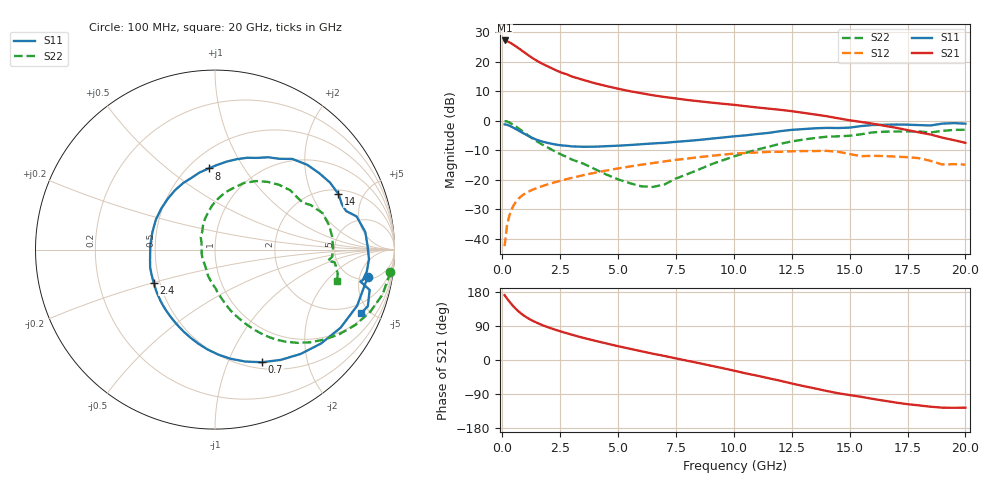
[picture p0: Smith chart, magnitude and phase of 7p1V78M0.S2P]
! Infineon Technologies  Discrete & RF Semiconductors
! bfp620
! VCE =  1.7 V,  IC =  8.0 mA
! Common Emitter S-Parameters:  Sep 2002
# GHz  S  MA  R  50
!  f  S11  S21  S12  S22
! GHz  MAG  ANG  MAG  ANG  MAG  ANG  MAG  ANG
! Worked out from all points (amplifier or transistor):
!   59 points, 100 MHz to 20 GHz, reference 50 ohm
!   highest |S21| = 27.1 dB at 100 MHz (marker M1)
!   |S21| within 3 dB of that: start of sweep to 769.9 MHz
!   unconditionally stable (mu >= 1): 4.315 GHz to 10.93 GHz; 17.11 GHz to end of sweep
!   at 1 GHz: K = 0.43, MSG = 23.7 dB, |S12| = -24.6 dB
!   at 5.5 GHz: K = 1.05, MAG = 11.5 dB, |S12| = -15.5 dB
!   at 20 GHz: K = 1.35, MAG = 0.1 dB, |S12| = -14.9 dB
!   S11 on the Smith chart (normalised r, x): 100 MHz: 5.47, -6.68; 700 MHz: 0.57, -1.34; 2.4 GHz: 0.46, -0.20; 8 GHz: 0.62, +0.71; 14 GHz: 2.23, +3.21; 20 GHz: 1.32, -4.43
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0.1  0.8642 -10.3  22.77 171.1  0.0075 80.8  0.9855 -7.3
0.2  0.8514 -21.6  22.17 162.5  0.0164 78.3  0.9666 -15.0
0.3  0.824 -31.9  21.26 154.6  0.0243 73.8  0.9315 -21.9
0.4  0.7893 -41.5  20.2 147.2  0.0312 69.4  0.8872 -28.3
0.5  0.7522 -50.6  19.07 140.4  0.0374 65.4  0.8389 -34.1
0.6  0.7155 -59.2  17.95 134.1  0.0428 61.9  0.7894 -39.4
0.7  0.6801 -67.3  16.86 128.4  0.0476 58.8  0.7407 -44.2
0.8  0.6464 -74.8  15.81 123.2  0.0518 56.1  0.6938 -48.5
1  0.5849 -88.3  13.88 114.4  0.059 51.7  0.6076 -55.7
1.2  0.5322 -100.1  12.22 107.1  0.0649 48.5  0.5332 -61.2
1.4  0.49 -110.6  10.86 100.9  0.07 46.2  0.4715 -65.7
1.9  0.4253 -132.9  8.529 88.0  0.0819 42.3  0.3618 -74.6
2.4  0.3884 -151.8  6.888 77.7  0.0934 39.4  0.2846 -81.3
3.5  0.3612 176.0  4.89 58.4  0.1195 32.9  0.1875 -95.3
5  0.377 142.4  3.469 36.4  0.1553 22.6  0.1013 -124.1
7  0.4209 108.0  2.516 10.7  0.204 6.8  0.0828 154.8
8  0.4534 94.5  2.234 -2.1  0.2281 -2.5  0.1245 124.6
10.5  0.5633 65.1  1.76 -35.1  0.2836 -29.1  0.2835 86.7
13.5  0.7415 30.3  1.272 -75.0  0.3059 -62.2  0.5077 45.3
14  0.7543 24.2  1.19 -81.6  0.3082 -68.7  0.5343 38.1
17  0.8595 -3.5  0.758 -112.3  0.2459 -93.1  0.6565 6.3
20  0.8882 -23.5  0.421 -125.8  0.1801 -105.3  0.702 -14.4
